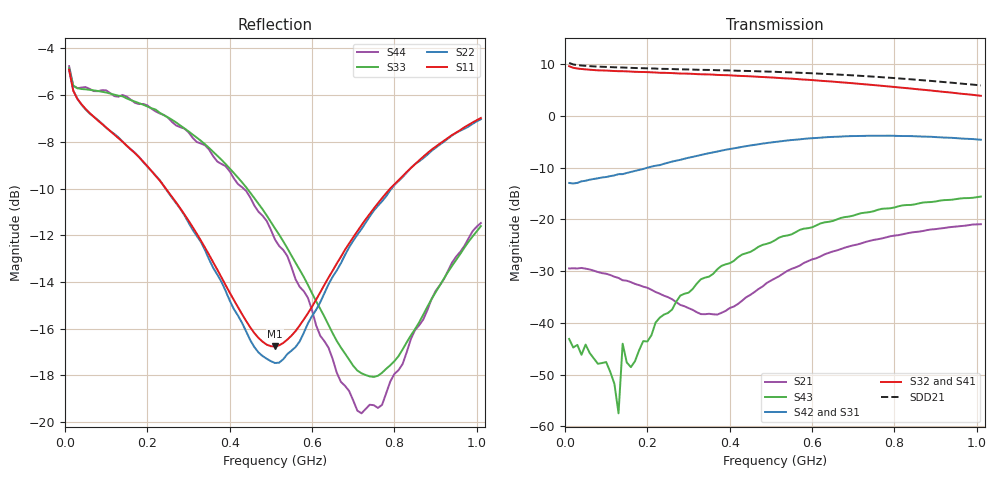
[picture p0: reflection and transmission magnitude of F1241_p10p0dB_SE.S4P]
! Integrated Device Technology
! Corporate Headquarters
! 6024 Silver Creek Valley Road
! San Jose, CA 95138  USA
! Phone:  1-408-284-8200
! Toll Free:  1-800-223-1366
! Webpage:  http://www.idt.com/
! Timing and RF Division
! 515 Groton Road, Suite 102
! Westford, MA 01886-6024
! Device:  F1241
! Description: Dual Intermediate Frequency Digital Variable Gain Amplifier
! Frequency:  10.0 -  500.00 MHz
! Package:  5x5 mm QFN Plastic Package: 32 pin
! Ports:  8 RF, 20 DC
!  Pin  1  = GA3  Pin 17  = RF OUT_B+
!  Pin  2  = GA4  Pin 18  = RF OUT_B-
!  Pin  3  = GA5  Pin 19  = STBY_B
!  Pin  4  = ISET_A  Pin 20  = Ground
!  Pin  5  = ISET_B  Pin 21  = Ground
!  Pin  6  = GB5  Pin 22  = STB_A
!  Pin  7  = GB4  Pin 23  = RF OUT_A-  = Port 4
!  Pin  8  = GB3  Pin 24  = RF OUT_A+  = Port 3
!  Pin  9  = GB2  Pin 25  = NO CONNECT
!  Pin 10  = GB1  Pin 26  = NO CONNECT
!  Pin 11  = RF IN_B+  Pin 27  = VCC
!  Pin 12  = RF IN_B-  Pin 28  = Ground
!  Pin 13  = Ground  Pin 29  = RF IN_A-  = Port 2
!  Pin 14  = VCC  Pin 30  = RF IN_A+  = Port 1
!  Pin 15  = NO CONNECT  Pin 31  = GA1
!  Pin 16  = NO CONNECT  Pin 32  = GA2
! State:  10
! Gain State:  10.0 dB
! Voltages:  Vcc = +5.00 Volts  Icc approximately 160.0 mA or 80 mA per channel.
! Data:  The device was measured on a custom evaluation board which has
!  individual transmission lines to the RF pins.  Data was collected
!  using a calibrated network analyzer.  The evaluation board was
!  de-embedded using a port reference technique.
!  The reference plane is the edge of the package pin.
!  Only Channel A was measured.
!  This data is in single-ended operation.  If your needs are balanced
!  or differential S-parameters then this file needs to be used a
!  linear simulator.
! Misc:  Lot Code  160028MY
!  Action Tracker AT004
! Date Measured:  2014-08-14
! Date:  2014-08-28  MJV
! Note:
!  Integrated Device Technology supplies this data as a sample of measured
!  data at the package pin for this product.  Your particular data for this
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# Hz S dB R 50
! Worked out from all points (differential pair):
!   101 points, 10 MHz to 1.01 GHz, reference 50 ohm
!   strongest paths, dB at 10 MHz, 260 MHz, 510 MHz, 760 MHz, 1.01 GHz:
!     S32: 9.6, 8.3, 7.4, 5.9, 3.9
!     S41: 9.6, 8.2, 7.3, 5.7, 3.7
!     S42: -13.0, -8.8, -5.0, -3.8, -4.6
!     S31: -13.0, -8.9, -5.1, -3.9, -4.7
!     S43: -43.1, -37.4, -24.0, -18.1, -15.6
!     S21: -29.5, -35.4, -31.4, -23.8, -20.9
!   taken as a pair (ports 2,1 in; 3,4 out), SDD21 dB: 10.2, 9.0, 8.5, 7.5, 5.9
!   lowest |S11| = -16.8 dB at 510 MHz (marker M1), VSWR 1.34, Z = 39.6 - j7.91 ohm
!   |S11| at or under -10 dB: 244.7 MHz to 789.8 MHz (545.1 MHz wide, 105 % of centre)
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1e7  -4.91 -18.7  -29.43 3.0  -52.34 49.7  -18.52 12.6
     -29.47 2.8  -4.92 -18.4  -18.55 12.3  -52.34 49.9
     -12.98 1.9  9.60 -179.8  -4.84 -16.6  -42.83 65.8
     9.62 -179.7  -12.96 2.0  -43.08 66.2  -4.76 -16.7
1.3e8  -7.84 -28.6  -31.29 -11.4  -37.88 63.6  -18.86 -7.4
       -31.31 -13.2  -7.81 -27.2  -18.85 -7.1  -38.01 63.1
       -11.30 11.7  8.63 159.7  -6.02 -13.8  -56.07 -6.1
       8.64 159.2  -11.26 11.5  -57.46 59.1  -6.06 -12.9
1.4e8  -8.00 -30.0  -31.72 -12.6  -37.15 63.7  -18.91 -7.9
       -31.76 -14.5  -7.99 -28.7  -18.87 -7.7  -37.14 63.5
       -11.29 10.5  8.62 158.2  -6.05 -14.9  -47.51 100.4
       8.61 157.6  -11.26 10.2  -44.01 97.4  -5.99 -14.1
3.7e8  -13.48 -76.7  -36.17 37.1  -29.66 44.0  -18.40 -18.7
       -38.38 36.0  -13.69 -72.9  -18.36 -18.5  -29.66 42.6
       -7.00 3.1  7.91 127.5  -8.60 -38.0  -31.17 124.7
       7.87 126.8  -6.89 2.2  -29.63 121.5  -8.84 -36.5
5.1e8  -16.76 -137.7  -30.76 66.0  -27.45 30.3  -18.05 -28.4
       -31.40 72.9  -17.47 -136.7  -17.92 -28.2  -27.42 28.4
       -5.15 -12.8  7.37 109.0  -11.71 -57.6  -25.01 109.9
       7.28 108.2  -5.05 -14.4  -24.03 105.9  -12.18 -55.6
7.2e8  -11.57 149.0  -24.71 57.3  -25.56 11.4  -18.03 -45.3
       -24.62 63.7  -11.74 147.7  -17.74 -45.5  -25.50 7.8
       -3.97 -41.5  6.15 82.1  -17.91 -122.1  -19.68 83.3
       6.01 81.3  -3.88 -43.9  -18.79 78.1  -19.63 -125.6
1.01e9  -6.98 117.6  -21.32 37.5  -24.25 -12.1  -19.02 -67.6
        -20.93 39.9  -7.03 117.0  -18.53 -68.1  -24.25 -16.7
        -4.74 -78.4  3.87 49.5  -11.61 151.8  -16.27 47.3
        3.68 48.8  -4.61 -81.8  -15.59 43.8  -11.48 145.8
